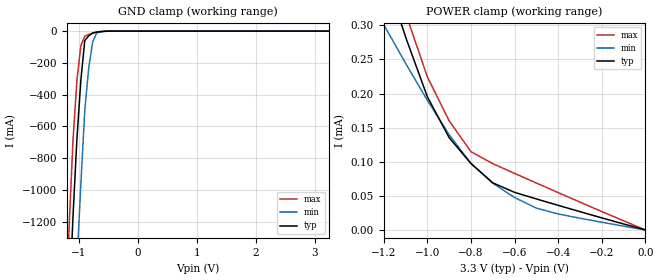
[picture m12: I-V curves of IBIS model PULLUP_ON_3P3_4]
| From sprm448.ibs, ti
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|BUFFER OPERATING IN WEAK PULLUP MODE
|   Model Cell PULLUP_ON_3P3
|PULLUP_ON_3P3
[Model]   PULLUP_ON_3P3_4
Model_type   Input
Polarity   Non-Inverting
Vinl =  0.8v
Vinh =  2v
C_comp   2.0027p   1.6434p   2.65p
[Model Spec]
Vinl   0.8v   0.8v   0.8v
Vinh   2v   2v   2v
[Temperature Range]   25   125   -40
[Voltage Range]   3.3   3   3.6
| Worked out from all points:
|   GND clamp passes 1 mA (typ) near -0.55 V on its own axis
|   POWER clamp passes 1 mA (typ) near -1.78 V on its own axis
[POWER_clamp]
|   voltage   I(typ)   I(min)   I(max)
-3.3V     2.699mA    1.574mA    4.071mA
-1.2V     381.8uA    301uA      459.6uA
-1.167V   348.8uA    282.2uA    412.4uA
-1.133V   315.9uA    263.3uA    365.2uA
-1.1V     282.9uA    244.5uA    317.9uA
-1.067V   253.6uA    226.3uA    286.7uA
-1V       195.2uA    190uA      224.3uA
-900mV    135.3uA    139.6uA    160uA
-800mV    97.36uA    97.54uA    114.7uA
-700mV    69.06uA    68.59uA    97.2uA
-500mV    45.48uA    32.08uA    68.8uA
-11.55fV  37.65pA    5.388nA    461.9fA
[GND_clamp]
|   voltage   I(typ)   I(min)   I(max)
-3.3V     -22.4A     -23.17A    -21.98A
-1.233V   -2.327A    -3.192A    -1.823A
-1.167V   -1.741A    -2.598A    -1.245A
-1.1V     -1.17A     -2.014A    -689.7mA
-1.033V   -680.3mA   -1.468A    -310.2mA
-966.7mV  -310.2mA   -963.5mA   -90.96mA
-900mV    -59.69mA   -500.1mA   -31.91mA
-833.3mV  -29.97mA   -231.2mA   -22.05mA
-766.7mV  -12.16mA   -68.65mA   -13.57mA
-700mV    -6.28mA    -12.31mA   -6.479mA
-433.3mV  -179uA     -296.9uA   -215.7uA
3.233V    -5.66uA    13.28uA    -45.87uA
